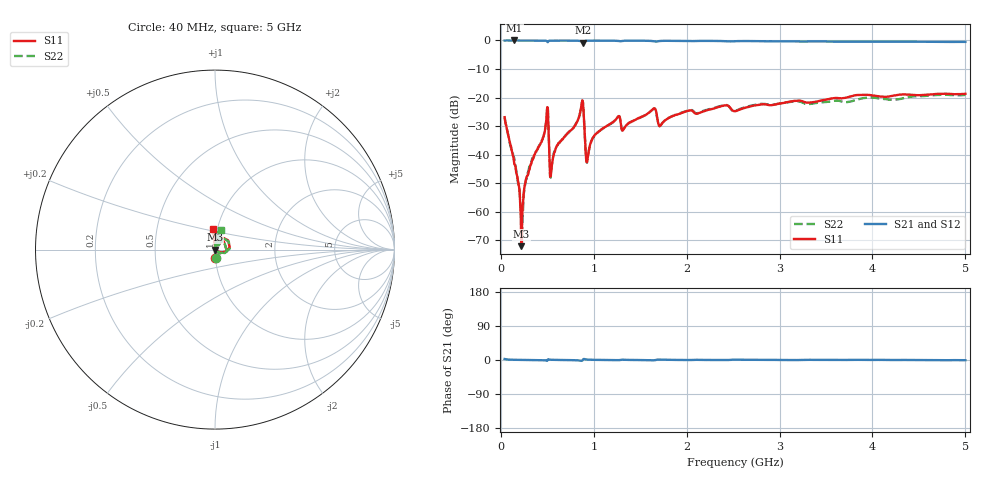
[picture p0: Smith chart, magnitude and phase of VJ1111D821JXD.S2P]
! VJ1111D821JXD
! DATE 02/15/2022  13:54
! CAPACITORS MOUNTED IN SERIES ON 25 MIL THICK MICROSTRIP SUBSTRATE
# GHz  S  MA  R  50.00
!  FREQ  S11M  S11A  S21M  S21A  S12M  S12A  S22M  S22A
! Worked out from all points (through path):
!   801 points, 40 MHz to 5 GHz, reference 50 ohm
!   highest |S21| = 0.01 dB at 145.4 MHz (marker M1); lowest = -0.8 dB at 883.2 MHz (marker M2)
!   lowest |S11| = -72.0 dB at 219.8 MHz (marker M3), VSWR 1.00, Z = 50 + j0.0101 ohm
!   |S11| at or under -10 dB: start of sweep to end of sweep
!   |S22| runs from -71.2 to -19.0 dB; largest |S21 - S12| = 0.011
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0.04  0.04542 -87.4  0.9981 2.7  0.9984 2.8  0.04555 -86.0
0.1454  0.006791 -86.2  1.001 0.8  0.9976 0.7  0.008479 -88.9
0.2198  0.0002501 23.8  0.9996 0.4  0.9997 0.2  0.0006682 -51.3
0.2384  0.001417 73.4  0.9994 0.3  0.9987 0.3  0.001087 74.1
0.257  0.002942 81.4  0.9988 0.1  0.9986 0.3  0.002742 77.1
0.2942  0.004555 86.1  0.9974 0.2  1 0.1  0.00505 80.0
0.4864  0.03714 77.0  0.9888 -1.3  0.9913 -1.1  0.03705 74.3
0.5484  0.006592 75.3  0.994 0.5  1 0.6  0.006549 71.7
0.6104  0.01473 88.2  0.995 0.1  1.001 0.3  0.01485 83.3
0.8708  0.08029 54.2  0.9471 -2.2  0.9517 -2.3  0.07945 48.9
0.8832  0.08281 8.8  0.9145 1.0  0.9196 1.0  0.08173 3.3
0.9328  0.008333 60.1  0.9912 1.1  0.9968 1.0  0.008387 56.4
1.0134  0.02251 88.5  0.9949 0.4  0.9979 0.3  0.02169 82.8
1.2552  0.045 82.9  0.9855 -0.4  0.9898 -0.5  0.04492 75.5
1.3234  0.02831 84.2  0.9885 0.6  0.9944 0.5  0.02863 75.7
1.6396  0.06364 78.3  0.9739 -0.7  0.9776 -0.9  0.06285 67.4
1.6954  0.03458 58.7  0.9704 1.3  0.9761 1.2  0.03366 48.9
2.0302  0.05948 89.6  0.9798 -0.1  0.9869 -0.2  0.06064 77.4
2.52  0.05762 87.2  0.9725 0.7  0.9788 0.6  0.05832 75.2
3.3508  0.08316 94.1  0.9633 0.4  0.9685 0.2  0.07857 78.4
4.1754  0.1047 93.3  0.9538 0.1  0.9623 -0.1  0.0923 76.1
5  0.1167 94.7  0.9453 -0.5  0.9509 -0.7  0.1117 73.0
